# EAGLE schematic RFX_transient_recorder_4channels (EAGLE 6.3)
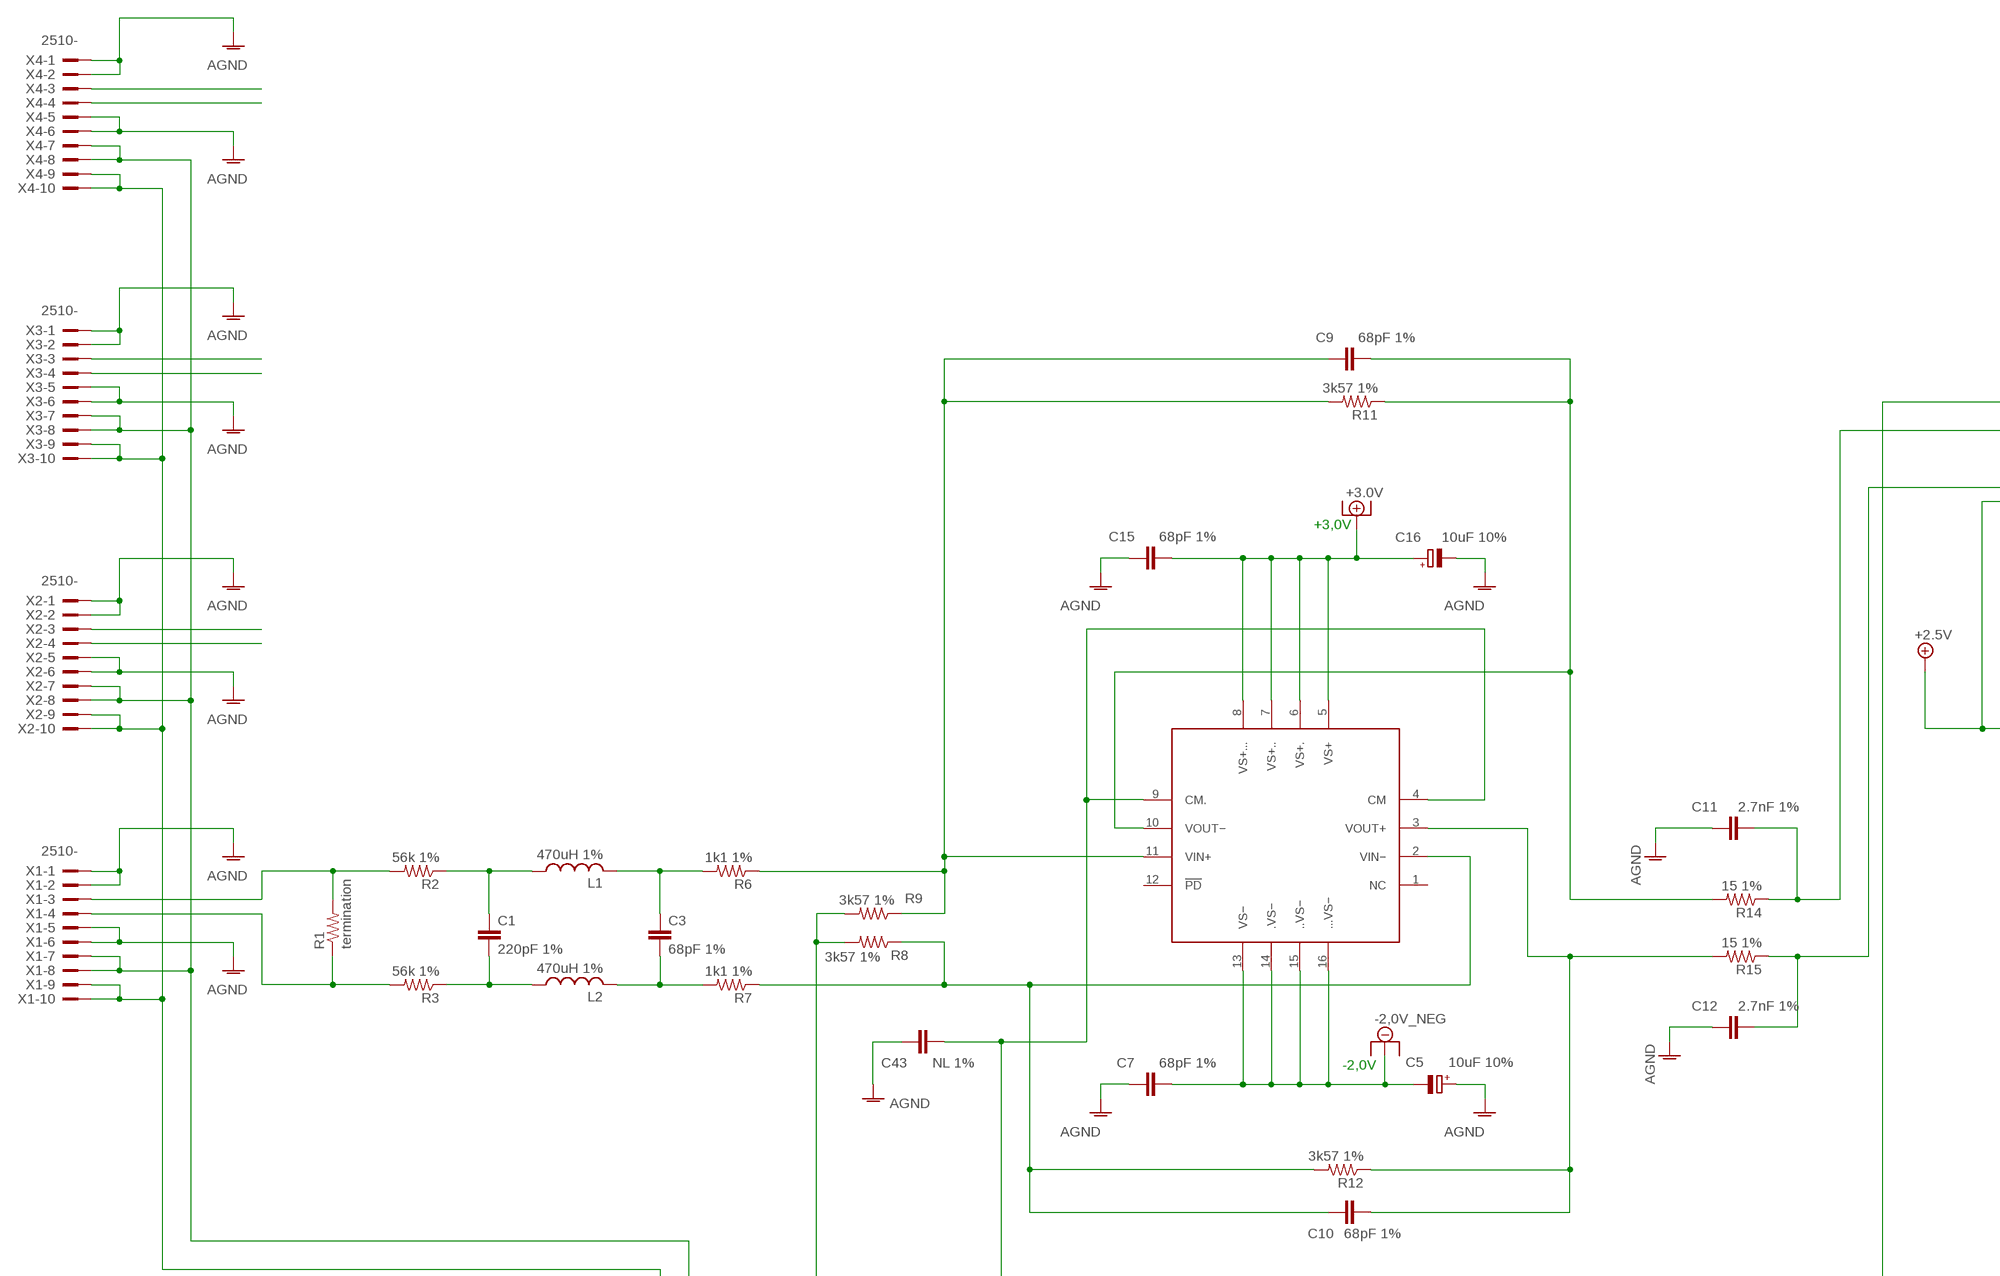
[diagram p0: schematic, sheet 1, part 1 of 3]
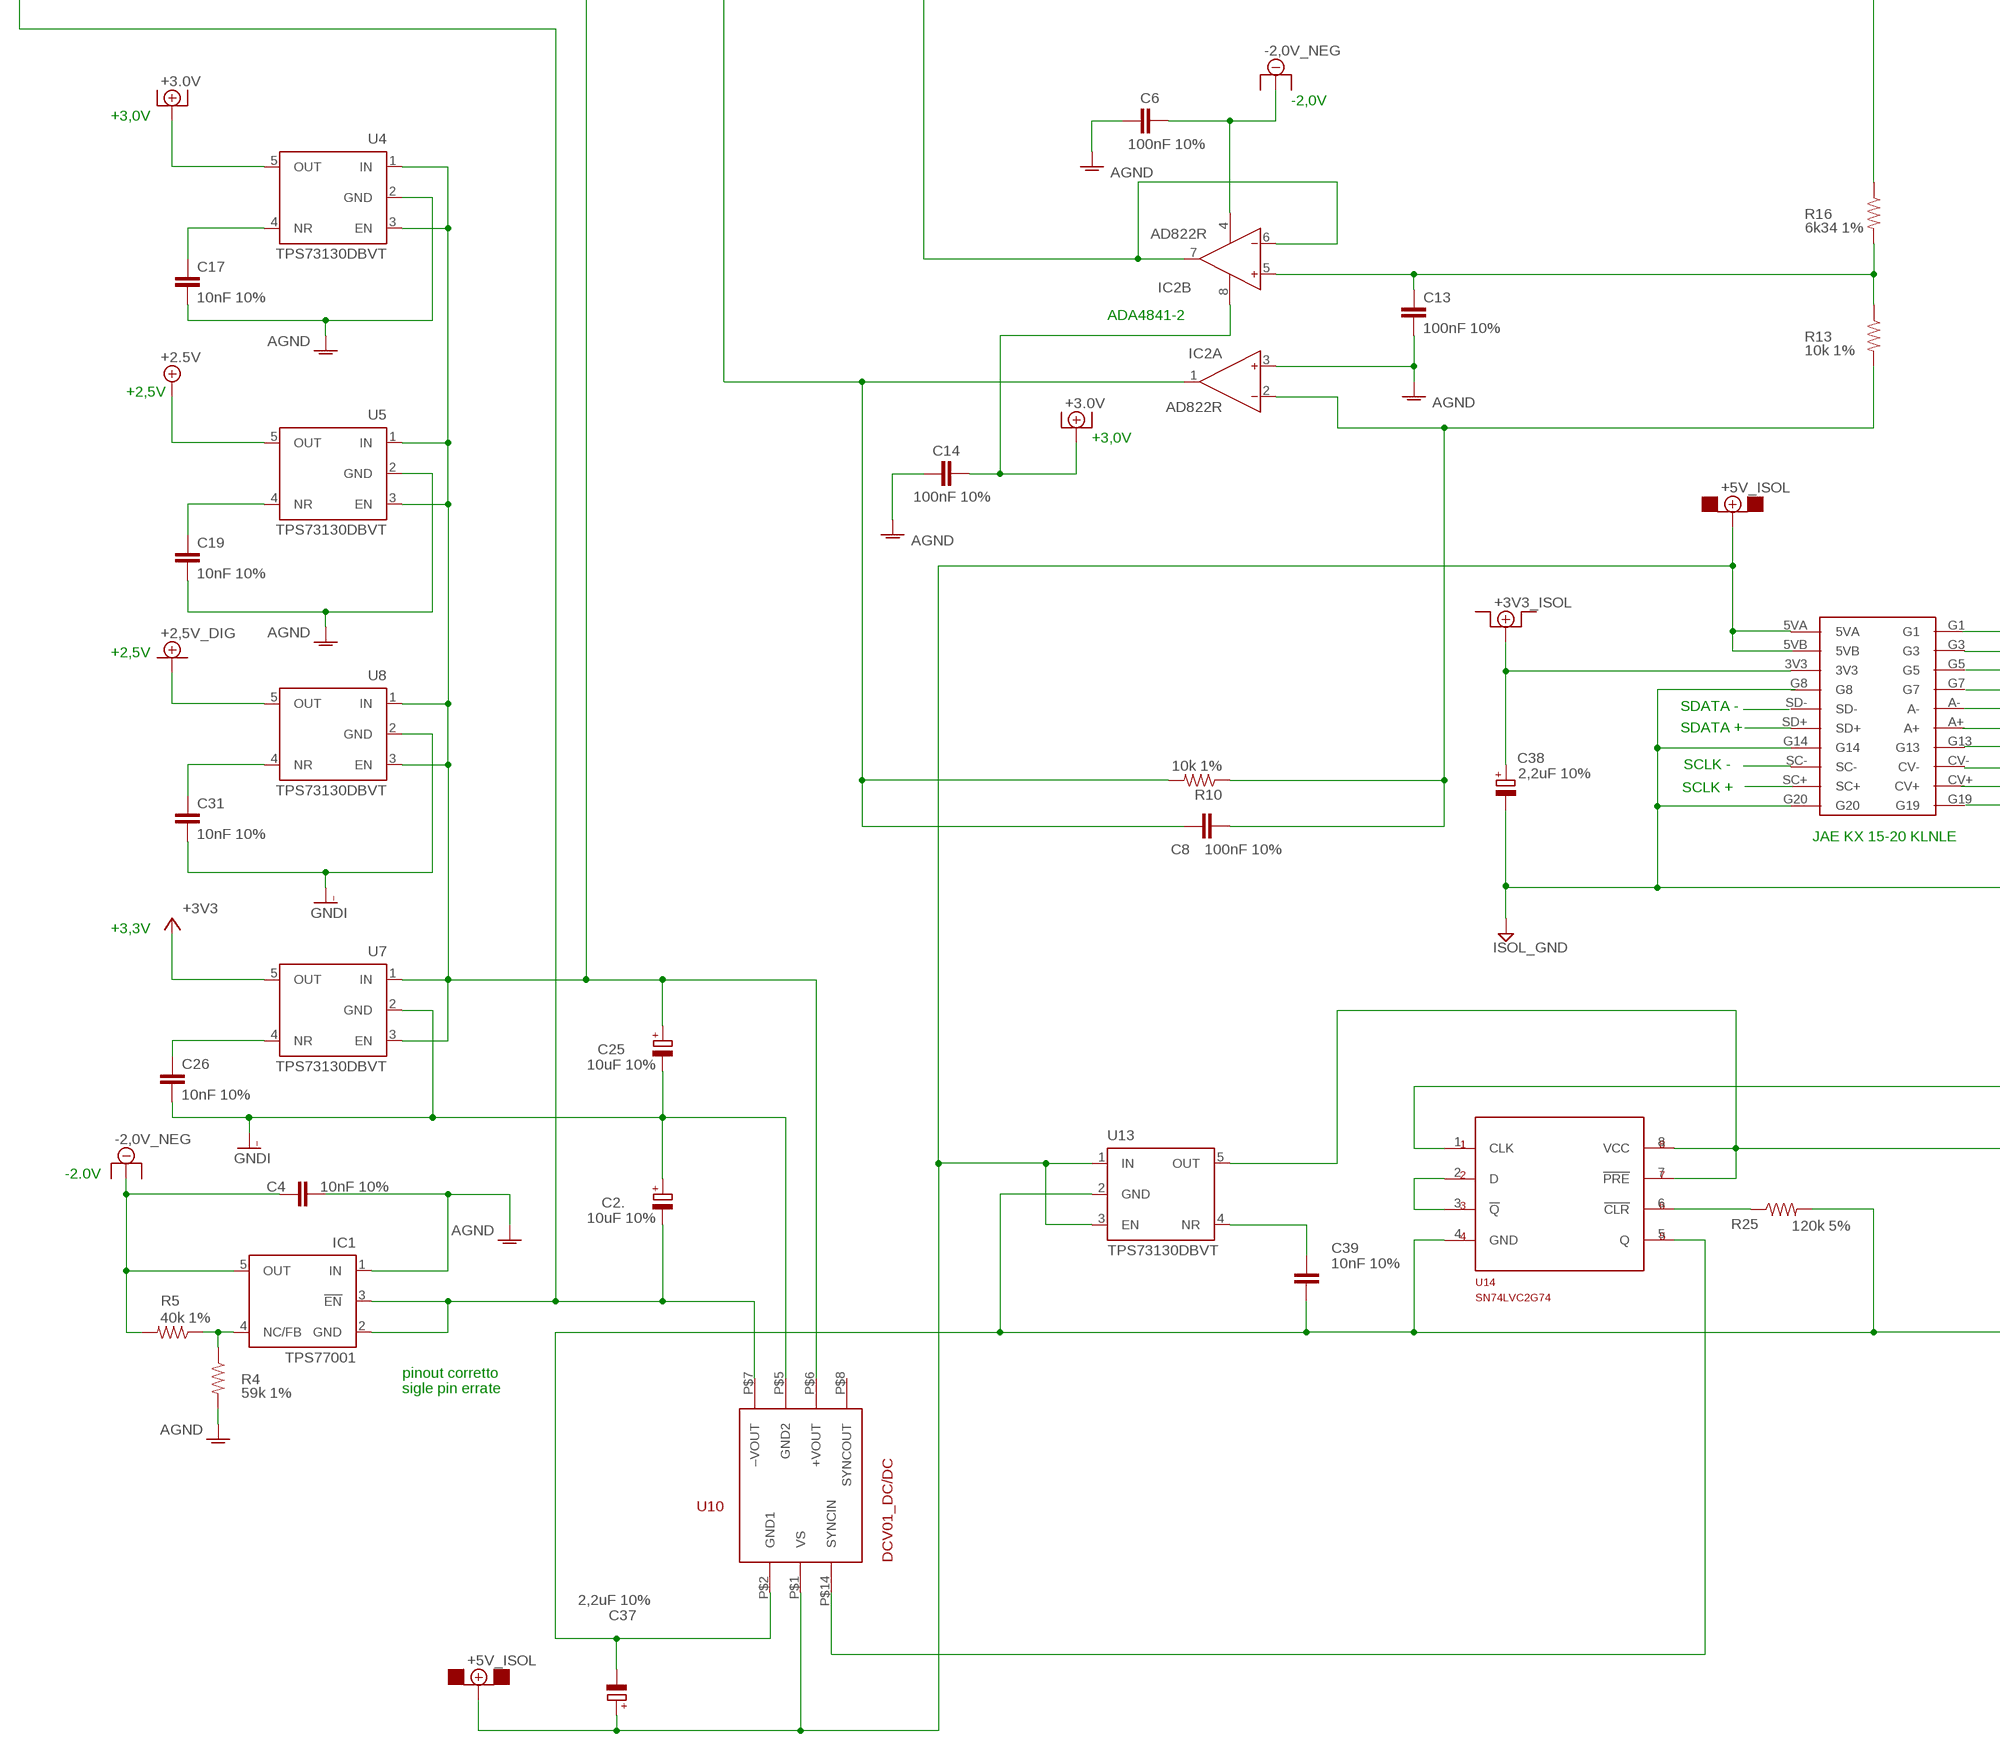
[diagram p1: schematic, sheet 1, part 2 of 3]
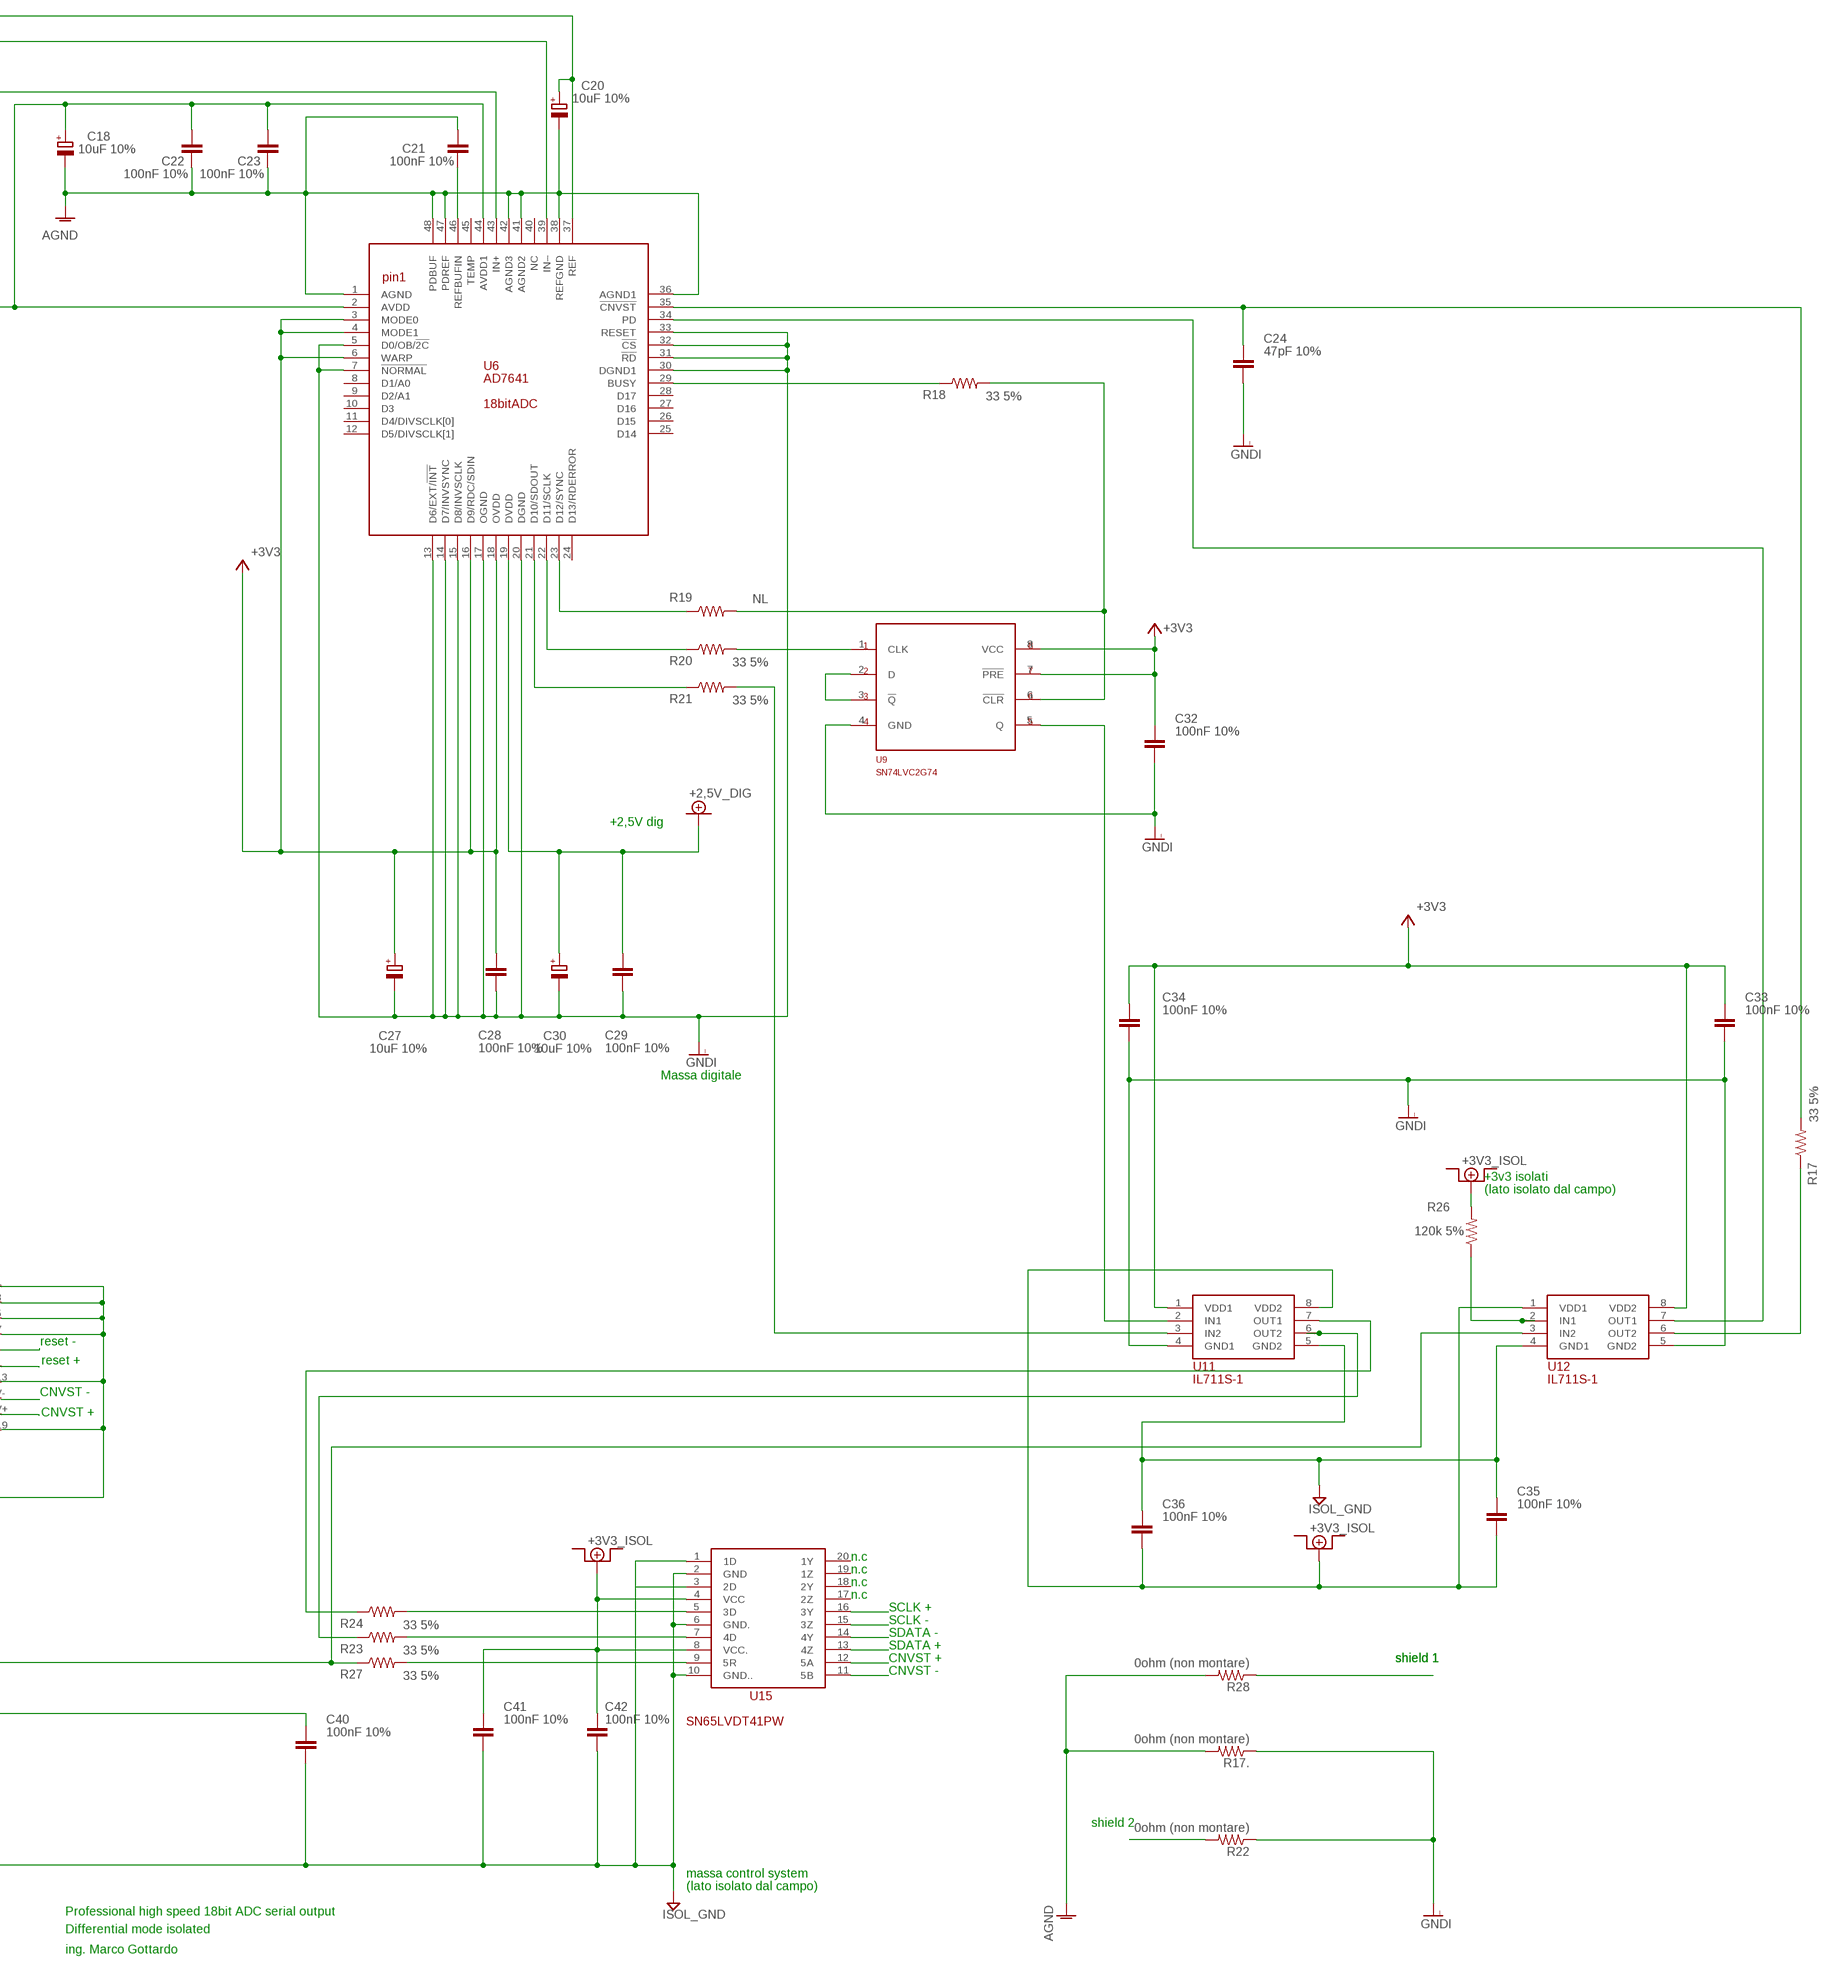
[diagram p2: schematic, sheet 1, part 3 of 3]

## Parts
C1  220pF 1%  C-EUC0805K  [C0805K]
C2.  10uF 10%  CPOL-EUSMCA  [SMC_A]
C3  68pF 1%  C-EUC0805K  [C0805K]
C4  10nF 10%  C-EUC0805K  [C0805K]
C5  10uF 10%  CPOL-EUSMCA  [SMC_A]
C6  100nF 10%  C-EUC0805K  [C0805K]
C7  68pF 1%  C-EUC0805K  [C0805K]
C8  100nF 10%  C-EUC0805K  [C0805K]
C9  68pF 1%  C-EUC0805K  [C0805K]
C10  68pF 1%  C-EUC0805K  [C0805K]
C11  2.7nF 1%  C-EUC0805K  [C0805K]
C12  2.7nF 1%  C-EUC0805K  [C0805K]
C13  100nF 10%  C-EUC0805K  [C0805K]
C14  100nF 10%  C-EUC0805K  [C0805K]
C15  68pF 1%  C-EUC0805K  [C0805K]
C16  10uF 10%  CPOL-EUSMCA  [SMC_A]
C17  10nF 10%  C-EUC0805K  [C0805K]
C18  10uF 10%  CPOL-EUSMCA  [SMC_A]
C19  10nF 10%  C-EUC0805K  [C0805K]
C20  10uF 10%  CPOL-EUSMCA  [SMC_A]
C21  100nF 10%  C-EUC0805K  [C0805K]
C22  100nF 10%  C-EUC0805K  [C0805K]
C23  100nF 10%  C-EUC0805K  [C0805K]
C24  47pF 10%  C-EUC0805K  [C0805K]
C25  10uF 10%  CPOL-EUSMCA  [SMC_A]
C26  10nF 10%  C-EUC0805K  [C0805K]
C27  10uF 10%  CPOL-EUSMCA  [SMC_A]
C28  100nF 10%  C-EUC0805K  [C0805K]
C29  100nF 10%  C-EUC0805K  [C0805K]
C30  10uF 10%  CPOL-EUSMCA  [SMC_A]
C31  10nF 10%  C-EUC0805K  [C0805K]
C32  100nF 10%  C-EUC0805K  [C0805K]
C33  100nF 10%  C-EUC0805K  [C0805K]
C34  100nF 10%  C-EUC0805K  [C0805K]
C35  100nF 10%  C-EUC0805K  [C0805K]
C36  100nF 10%  C-EUC0805K  [C0805K]
C37  2,2uF 10%  CPOL-EUSMCA  [SMC_A]
C38  2,2uF 10%  CPOL-EUSMCA  [SMC_A]
C39  10nF 10%  C-EUC0805K  [C0805K]
C40  100nF 10%  C-EUC0805K  [C0805K]
C41  100nF 10%  C-EUC0805K  [C0805K]
C42  100nF 10%  C-EUC0805K  [C0805K]
C43  NL 1%  C-EUC0805K  [C0805K]
IC1  TPS77001  [SOT23-DBV]
IC2  AD822R  [SO8]
L1  470uH 1%  L-USL3216C  [L3216C]
L2  470uH 1%  L-USL3216C  [L3216C]
R1  termination  R-US_R0402  [R0402]
R2  56k 1%  R-US_R0402  [R0402]
R3  56k 1%  R-US_R0402  [R0402]
R4  59k 1%  R-US_R0402  [R0402]
R5  40k 1%  R-US_R0402  [R0402]
R6  1k1 1%  R-US_R0402  [R0402]
R7  1k1 1%  R-US_R0402  [R0402]
R8  3k57 1%  R-US_R0402  [R0402]
R9  3k57 1%  R-US_R0402  [R0402]
R10  10k 1%  R-US_R0402  [R0402]
R11  3k57 1%  R-US_R0402  [R0402]
R12  3k57 1%  R-US_R0402  [R0402]
R13  10k 1%  R-US_R0402  [R0402]
R14  15 1%  R-US_R0402  [R0402]
R15  15 1%  R-US_R0402  [R0402]
R16  6k34 1%  R-US_R0402  [R0402]
R17  33 5%  R-US_R0402  [R0402]
R17.  0ohm (non montare)  R-US_R0402  [R0402]
R18  33 5%  R-US_R0402  [R0402]
R19  NL  R-US_R0402  [R0402]
R20  33 5%  R-US_R0402  [R0402]
R21  33 5%  R-US_R0402  [R0402]
R22  0ohm (non montare)  R-US_R0402  [R0402]
R23  33 5%  R-US_R0402  [R0402]
R24  33 5%  R-US_R0402  [R0402]
R25  120k 5%  R-US_R0402  [R0402]
R26  120k 5%  R-US_R0402  [R0402]
R27  33 5%  R-US_R0402  [R0402]
R28  0ohm (non montare)  R-US_R0402  [R0402]
U4  TPS73130DBVT  [SOT23-DBV]
U5  TPS73130DBVT  [SOT23-DBV]
U6  AD7641  [QFP-7X7-48]
U7  TPS73130DBVT  [SOT23-DBV]
U8  TPS73130DBVT  [SOT23-DBV]
U9  SN74LVC2G74  [SO-08]
U10  DCV01_DC/DCDCV010505DP_DC/DC_CONVERTER  [DCV10_DC/DC]
U11  IL711S-1  [SO-08]
U12  IL711S-1  [SO-08]
U13  TPS73130DBVT  [SOT23-DBV]
U14  SN74LVC2G74  [SO-08]
U15  SN65LVDT41PW  [TSSOP16]
U$1  THS4520_QFN16  [QFN16]
U$20  JAE-CONNECTOR  [JAECONNECTOR]
X1  2510-  [PAK100/2500-10]
X2  2510-  [PAK100/2500-10]
X3  2510-  [PAK100/2500-10]
X4  2510-  [PAK100/2500-10]

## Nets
+2.5V: C18.+ C22.2 C23.2 U5.5(OUT) U6.2(AVDD) U6.44(AVDD1)
+2.5V_DIG: C29.2 C30.+ U6.19(DVDD) U8.5(OUT) ; supply symbol labelled +2,5V_DIG
+3.0V: C14.2 C15.2 C16.+ IC2.8(P:V+) U4.5(OUT) U$1.5(VS+) U$1.6(VS+.) U$1.7(VS+..) U$1.8(VS+...)
+3V3: C27.+ C28.2 C32.2 C33.2 C34.2 U6.3(MODE0) U6.4(MODE1) U6.6(WARP) U6.16(D9/RDC/SDIN) U6.18(OVDD) U7.5(OUT) U9.7(!PRE!) U9.8(VCC) U11.1(VDD1) U12.8(VDD2)
+3V3_ISOL: C35.1 C36.1 C38.+ C41.2 C42.2 R26.2 U11.8(VDD2) U12.1(VDD1) U15.4(VCC) U15.8(VCC.)
+5V_ISOL: C37.+ U10.P$1(VS) U13.1(IN) U13.3(EN)
-2.0V_NEG: C4.1 C5.- C6.2 C7.2 IC1.5(OUT) IC2.4(P:V-) R5.2 U$1.13(VS−) U$1.14(.VS−) U$1.15(..VS−) U$1.16(...VS−) ; supply symbol labelled -2,0V_NEG
AGND: C4.2 C5.+ C6.1 C7.1 C11.1 C12.1 C13.2 C14.1 C15.1 C16.- C17.2 C18.- C19.2 C20.- C21.2 C22.1 C23.1 C43.1 IC1.1(IN) IC2.3(A:IN+) R4.2 R17..2 R28.2 U4.2(GND) U5.2(GND) U6.1(AGND) U6.36(AGND1) U6.38(REFGND) U6.41(AGND2) U6.42(AGND3) U6.47(PDREF) U6.48(PDBUF) X1.1 X1.2 X1.5 X1.6 X2.1 X2.2 X2.5 X2.6 X3.1 X3.2 X3.5 X3.6 X4.1 X4.2 X4.5 X4.6
GNDI: C2..+ C24.1 C25.- C26.2 C27.- C28.1 C29.1 C30.- C31.2 C32.1 C33.1 C34.1 R17..1 R22.1 U6.5(D0/OB/!2C!) U6.7(!NORMAL!) U6.13(D6/EXT/!INT!) U6.14(D7/INVSYNC) U6.15(D8/INVSCLK) U6.17(OGND) U6.20(DGND) U6.30(DGND1) U6.31(!RD!) U6.32(!CS!) U6.33(RESET) U7.2(GND) U8.2(GND) U9.4(GND) U10.P$5(GND2) U11.4(GND1) U12.5(GND2)
ISOL_GND: C35.2 C36.2 C37.- C38.- C39.1 C40.1 C41.1 C42.1 R25.2 U10.P$2(GND1) U11.5(GND2) U12.4(GND1) U13.2(GND) U14.4(GND) U15.1(1D) U15.2(GND) U15.3(2D) U15.6(GND.) U15.10(GND..)
N$1: C3.1 L1.2 R6.2
N$2: C1.1 L1.1 R2.1
N$3: C3.2 L2.2 R7.2
N$4: C1.2 L2.1 R3.1
N$5: C9.1 R6.1 R9.1 R11.2 U$1.11(VIN+)
N$6: C10.1 R7.1 R8.1 R12.2 U$1.2(VIN−)
N$7: R20.2 U9.1(CLK)
N$8: R1.2 R2.2 X1.3
N$9: R1.1 R3.2 X1.4
N$10: C9.2 R11.1 R14.2 U$1.10(VOUT−)
N$11: C10.2 R12.1 R15.2 U$1.3(VOUT+)
N$12: C11.2 R14.1 U6.39(IN–)
N$13: C12.2 R15.1 U6.43(IN+)
N$14: R28.1
N$15: R22.2
N$16: C2..- IC1.2(GND) IC1.3(!EN) U10.P$7(–VOUT) X1.9 X1.10 X2.9 X2.10 X3.9 X3.10 X4.9 X4.10
N$17: C17.1 U4.4(NR)
N$18: C25.+ U4.1(IN) U4.3(EN) U5.1(IN) U5.3(EN) U7.1(IN) U7.3(EN) U8.1(IN) U8.3(EN) U10.P$6(+VOUT) X1.7 X1.8 X2.7 X2.8 X3.7 X3.8 X4.7 X4.8
N$19: X2.3
N$20: C19.1 U5.4(NR)
N$21: X2.4
N$22: U15.16(3Y)
N$23: C31.1 U8.4(NR)
N$25: X3.3
N$26: C26.1 U7.4(NR)
N$27: IC1.4(NC/FB) R4.1 R5.1
N$28: C43.2 IC2.6(B:IN-) IC2.7(B:OUT) U$1.4(CM) U$1.9(CM.)
N$29: X3.4
N$30: C13.1 IC2.5(B:IN+) R13.1 R16.2
N$31: R20.1 U6.22(D11/SCLK)
N$32: C20.+ R16.1 U6.37(REF)
N$33: C21.1 U6.46(REFBUFIN)
N$34: U15.15(3Z)
N$35: U15.14(4Y)
N$36: R19.1 U6.23(D12/SYNC)
N$37: R18.2 R19.2 U9.6(!CLR!)
N$38: R18.1 U6.29(BUSY)
N$39: U9.2(D) U9.3(!Q!)
N$40: C8.1 IC2.1(A:OUT) R8.2 R9.2 R10.2
N$41: C8.2 IC2.2(A:IN-) R10.1 R13.2
N$42: U9.5(Q) U11.2(IN1)
N$43: R21.1 U6.21(D10/SDOUT)
N$44: R21.2 U11.3(IN2)
N$45: C24.2 R17.2 U6.35(!CNVST!)
N$46: R17.1 U12.6(OUT2)
N$47: U6.34(PD) U12.7(OUT1)
N$48: X4.3
N$49: X4.4
N$50: R27.1 U12.3(IN2) U14.1(CLK)
N$51: R24.2 U15.5(3D)
N$52: R23.2 U15.7(4D)
N$53: R24.1 U11.7(OUT1)
N$54: R23.1 U11.6(OUT2)
N$56: R27.2 U15.9(5R)
N$57: R26.1 U12.2(IN1)
N$58: U15.13(4Z)
N$59: U14.2(D) U14.3(!Q!)
N$60: R25.1 U14.6(!CLR!)
N$61: U10.P$14(SYNCIN) U14.5(Q)
N$62: C40.2 U13.5(OUT) U14.7(!PRE!) U14.8(VCC)
N$63: U15.12(5A)
N$64: C39.2 U13.4(NR)
N$65: U15.11(5B)
Unconnected: U6.8(D1/A0) U6.9(D2/A1) U6.10(D3) U6.11(D4/DIVSCLK[0]) U6.12(D5/DIVSCLK[1]) U6.24(D13/RDERROR) U6.25(D14) U6.26(D15) U6.27(D16) U6.28(D17) U6.40(NC) U6.45(TEMP) U10.P$8(SYNCOUT) U15.17(2Z) U15.18(2Y) U15.19(1Z) U15.20(1Y) U$1.1(NC) U$1.12(!PD!) U$20.3V3 U$20.5VA U$20.5VB U$20.A+ U$20.A- U$20.CV+ U$20.CV- U$20.G1 U$20.G3 U$20.G5 U$20.G7 U$20.G8 U$20.G13 U$20.G14 U$20.G19 U$20.G20 U$20.SC+ U$20.SC- U$20.SD+ U$20.SD-

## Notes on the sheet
- +3,0V
- -2,0V
- +2,5V dig
- -2,0V
- +3,0V
- ADA4841-2
- Massa digitale
- +2,5V
- +3,0V
- +3v3 isolati
- (lato isolato dal campo)
- +2,5V
- reset -
- SDATA -
- reset +
- SDATA +
- CNVST -
- SCLK -
- SCLK + | CNVST +
- JAE KX 15-20 KLNLE
- +3,3V
- n.c
- n.c
- n.c
- n.c
- SCLK +
- SCLK -
- SDATA -
- SDATA +
- CNVST + | shield 1 | shield 1
- CNVST -
- -2.0V
- shield 2
- massa control system
- (lato isolato dal campo)
- pinout corretto
- sigle pin errate | Professional high speed 18bit ADC serial output
- Differential mode isolated
- ing. Marco Gottardo

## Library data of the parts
C1 C3 C4 C6-C15 C17 C19 C21-C24 C26 C28 C29 C31-C36 C39-C43 = resistor:C-EU: CAPACITOR, European symbol
C2. C5 C16 C18 C20 C25 C27 C30 C37 C38 = resistor:CPOL-EU: POLARIZED CAPACITOR, European symbol
IC1 = texas:TPS770*: ULTRALOW-POWER 50-mA LOW-DROPOUT LINEAR REGULATORS 50-mA Low-Dropout Regulator Source: http://focus.ti.com/lit/ds/symlink/tps77001.pdf; MF: TEXAS INSTRUMENTS; MPN: TPS77001DBVT; OC_FARNELL: 8461554; OC_NEWARK: 77C1171
IC2 = analog-devices:AD822: Single-Supply, Rail-to-Rail Low Power FET-Input Op Amp Source: http://www.analog.com/static/imported-files/data_sheets/AD822.pdf; MF: ANALOG DEVICES; MPN: AD822BRZ; OC_FARNELL: 1651303
L1 L2 = resistor:L-US: INDUCTOR, American symbol
R1-R17 R17. R18-R28 = resistor:R-US_: RESISTOR, American symbol
U4 U5 U7 U8 U13 = TPS73130DBVT:TPS73130DBVT
U6 = AD7641:AD7641
U9 U14 = SN74LVC2G74DCUR_SOP8:SN74LVC2G74
U10 = DCV01_DCDC:DCV01_DC/DC
U11 U12 = IL711S-1 SOIC8:IL711S-1
U15 = SN65LVDT41PW-TSSOP20:SN65LVDT41PW: MEMORY STICK™ INTERCONNECT EXTENDER CHIPSET WITH LVDS
U$1 = THS4520 QFN16:THS4520_QFN16
U$20 = JAE-connector:JAE-CONNECTOR
X1-X4 = con-3m:2510-: 3M (TM) Pak 100 4-Wall Header Source: 3M; MF: 3M; MPN: 2510-6002UB; OC_FARNELL: 9838244; OC_NEWARK: 46F4725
